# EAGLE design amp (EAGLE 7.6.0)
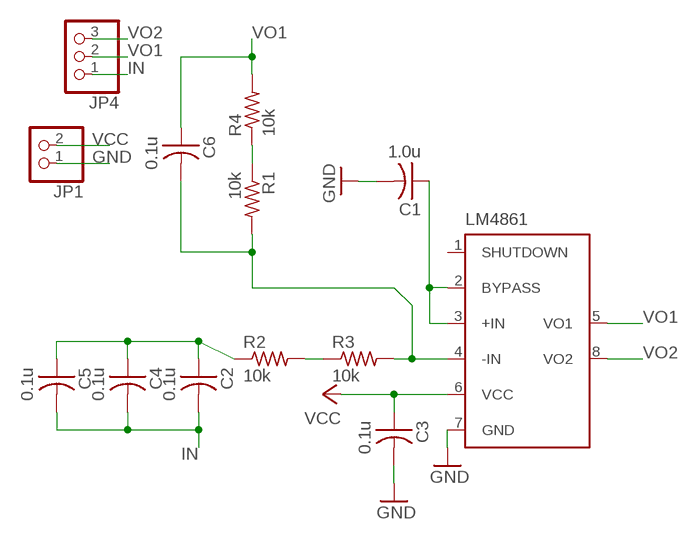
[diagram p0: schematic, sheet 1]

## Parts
C1  1.0u  CAP-US1206FAB  [C1206FAB]
C2  0.1u  CAP-US1206FAB  [C1206FAB]
C3  0.1u  CAP-US1206FAB  [C1206FAB]
C4  0.1u  CAP-US1206FAB  [C1206FAB]
C5  0.1u  CAP-US1206FAB  [C1206FAB]
C6  0.1u  CAP-US1206FAB  [C1206FAB]
IC1  MC1350  [SO08]
JP1  PINHD-1X2  [1X02]
JP4  PINHD-1X3  [1X03]
R1  10k  RES-US1206FAB  [R1206FAB]
R2  10k  RES-US1206FAB  [R1206FAB]
R3  10k  RES-US1206FAB  [R1206FAB]
R4  10k  RES-US1206FAB  [R1206FAB]

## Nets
GND: C1.2 C3.2 IC1.7(GND) JP1.1
IN: C2.2 C4.2 C5.2 JP4.1
N$1: C1.1 IC1.2(BYPASS) IC1.3(+IN)
N$2: C6.2 IC1.4(-IN) R1.2 R3.2
N$3: C2.1 C4.1 C5.1 R2.1
N$4: R2.2 R3.1
N$5: R1.1 R4.1
VCC: C3.1 IC1.6(VCC) JP1.2
VO1: C6.1 IC1.5(VO1) JP4.2 R4.2
VO2: IC1.8(VO2) JP4.3

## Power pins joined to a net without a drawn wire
SHUTDOWN: IC1.1(SHUTDOWN)

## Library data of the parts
C1-C6 = fab:CAP-US
IC1 = linear:MC1350: Monolitic IF Amplifier Source: MOTOROLA .. MC1350.pdf
JP1 = pinhead:PINHD-1X2: PIN HEADER
JP4 = pinhead:PINHD-1X3: PIN HEADER
R1-R4 = fab:RES-US: Resistor (US Symbol)

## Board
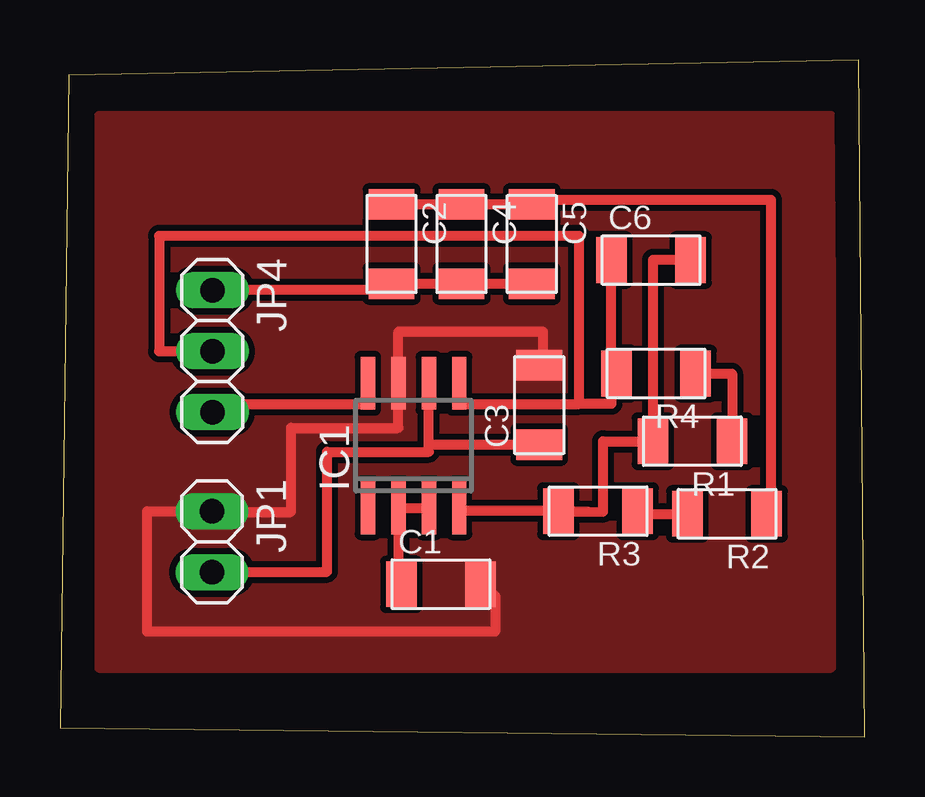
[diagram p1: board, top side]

Size 33.52 x 28.21 mm. Coordinates in mm from the lower left corner, seen from the top.
Outline: 0,0.37 33.52,0 33.28,28.21 0.37,27.59 0,0.37
Copper layers (1*16): Top 0.035mm / dielectric 1.5mm / Bottom 0.035mm
Design rules "default": minimum track width 10mil, minimum drill 24mil, track to track 8mil, track to pad 8mil, pad to pad 8mil, via to via 8mil, smd to smd 8mil, copper to edge 40mil, drill to drill 8mil, minimum pad ring 10mil, minimum via ring 8mil, stop-mask expansion 4mil, vias tented up to drill 0mil, thermal gap 10mil

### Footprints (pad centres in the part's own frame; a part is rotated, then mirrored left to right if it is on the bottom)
C1206FAB = smd 1.27 x 1.905: 1 -1.651,0; 2 1.651,0
SO08 = smd 0.6 x 2.2: 1 -1.905,-2.6; 2 -0.635,-2.6; 3 0.635,-2.6; 4 1.905,-2.6; 5 1.905,2.6; 6 0.635,2.6; 7 -0.635,2.6; 8 -1.905,2.6
1X02 = drill 1.016 long: 1 -1.27,0; 2 1.27,0
1X03 = drill 1.016 long: 1 -2.54,0; 2 0,0; 3 2.54,0
R1206FAB = smd 1.27 x 1.905: 1 -1.651,0; 2 1.651,0

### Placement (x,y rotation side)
C1  15.87,6.36 0 top
C2  13.81,20.54 270 top
C3  19.97,13.83 90 top
C4  16.73,20.54 270 top
C5  19.65,20.54 270 top
C6  24.63,19.87 0 top
IC1  14.73,12.14 0 top
JP1  6.33,8.13 270 top
JP4  6.35,16.07 270 top
R1  26.35,12.32 180 top
R2  27.8,9.29 180 top
R3  22.42,9.41 180 top
R4  24.84,15.14 180 top

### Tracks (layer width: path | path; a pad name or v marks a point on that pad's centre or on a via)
GND
  Top 0.406: C3.2 19.97,15.37 20.13,15.37 20.13,16.87 14.1,16.87 IC1.7 14.1,12.87 9.63,12.87 9.63,9.37 6.63,9.37 6.63,9.4 JP1.1 3.63,9.4 3.63,4.37 18.13,4.37 18.13,5.87 17.52,5.87 C1.2
  pour Top (isolate 0.254, no thermals): 1.63,25.87 1.63,2.87 32.13,2.87 32.13,25.87
IN
  Top 0.406: JP4.1 13.81,18.61 C2.2 C4.2 C5.2
N$1
  Top 0.406: IC1.3 IC1.2 14.1,6.36 C1.1
N$2
  Top 0.406: IC1.4 16.64,9.41 R3.2 arc-2 22.63,9.37 22.63,12.32 R1.2 24.7,19.87 C6.2 26.63,19.87
N$3
  Top 0.406: C2.1 C4.1 C5.1 19.65,22.37 29.63,22.37 29.63,9.29 R2.1
N$4
  Top 0.406: R3.1 24.07,9.29 R2.2
N$5
  Top 0.406: R4.1 28,15.14 R1.1
VCC
  Top 0.406: JP1.2 6.33,6.87 11.13,6.87 11.13,11.87 15.37,11.87 15.37,12.18 | 15.37,12.18 IC1.6 | 15.37,12.18 C3.1
VO1
  Top 0.406: R4.2 22.98,15.14 | 22.98,15.14 C6.1 | 22.98,15.14 22.98,13.87 21.63,13.87 | 21.63,13.87 21.63,20.87 4.13,20.87 4.13,16.07 JP4.2 | IC1.5 16.64,13.87 21.63,13.87
VO2
  Top 0.406: JP4.3 6.63,13.53 6.63,13.87 12.83,13.87 IC1.8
